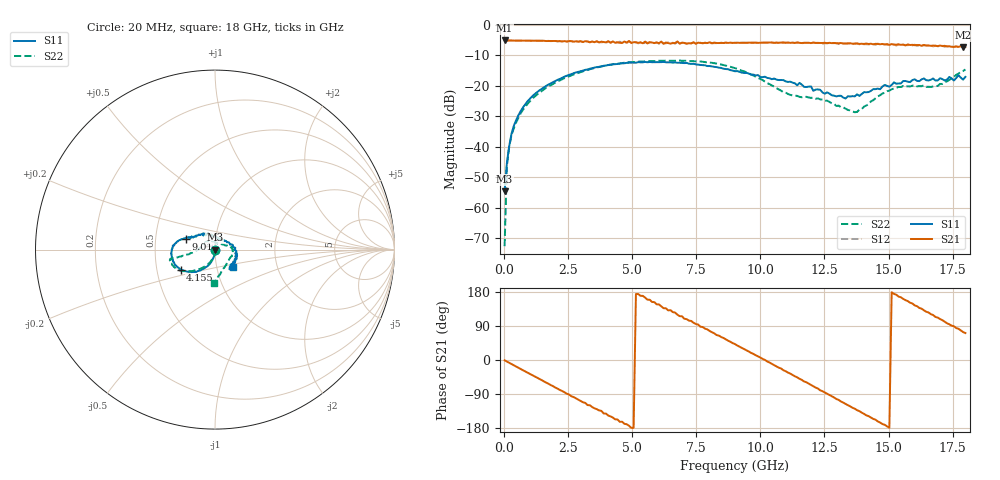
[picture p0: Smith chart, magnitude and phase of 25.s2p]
!Agilent Technologies,N5230A,US43500223,A.07.50.48
!Agilent N5230A: A.07.50.48
!Date: Wednesday, January 13, 2016 12:40:09
!Correction: S11(Full 2 Port(1,2))
!S21(Full 2 Port(1,2))
!S12(Full 2 Port(1,2))
!S22(Full 2 Port(1,2))
!S2P File: Measurements: S11, S21, S12, S22:
# Hz S  dB  R 50
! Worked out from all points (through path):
!   201 points, 20 MHz to 18 GHz, reference 50 ohm
!   highest |S21| = -5.16 dB at 20 MHz (marker M1); lowest = -7.4 dB at 17.91 GHz (marker M2)
!   group delay of S21, straight-line fit = 99.6 ps
!   lowest |S11| = -54.5 dB at 20 MHz (marker M3), VSWR 1.00, Z = 49.8 - j0.109 ohm
!   |S11| at or under -10 dB: start of sweep to end of sweep
!   |S22| runs from -72.5 to -11.7 dB; largest |S21 - S12| = 0.042
!   S11 on the Smith chart (normalised r, x): 20 MHz: 1.00, -0.00; 4.155 GHz: 0.66, -0.16; 9.01 GHz: 0.72, +0.09; 18 GHz: 1.20, -0.24
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2e7  -54.55 -144.2  -5.16 -0.8  -5.17 -0.9  -72.52 -110.8
1.099e8  -45.22 -107.3  -5.18 -4.1  -5.18 -4.1  -46.16 -82.0
2.897e8  -35.69 -91.2  -5.19 -10.8  -5.20 -10.8  -36.11 -87.4
4.695e8  -31.26 -95.9  -5.21 -17.2  -5.21 -17.4  -32.03 -93.7
9.19e8  -25.03 -103.3  -5.23 -33.6  -5.25 -33.8  -25.88 -103.0
1.3685e9  -21.57 -109.7  -5.29 -49.9  -5.29 -50.2  -22.32 -111.8
2.3574e9  -17.01 -124.9  -5.37 -85.2  -5.42 -85.5  -17.49 -127.2
3.0766e9  -15.04 -134.9  -5.69 -111.5  -5.61 -112.0  -15.25 -136.3
4.1554e9  -13.09 -149.8  -5.91 -148.9  -5.88 -150.2  -13.10 -147.9
4.8746e9  -12.43 -159.3  -5.33 -173.6  -5.57 -173.4  -12.29 -154.1
6.0433e9  -12.27 -173.6  -6.06 146.5  -6.28 143.8  -11.81 -162.9
7.3918e9  -12.82 172.7  -5.76 98.2  -5.83 97.9  -11.94 -168.2
9.01e9  -15.24 159.2  -5.92 42.0  -5.93 39.8  -14.24 -168.6
1.04484e10  -17.85 145.9  -5.81 -10.3  -5.90 -12.5  -19.90 -177.7
1.20666e10  -21.66 109.3  -5.83 -69.1  -5.97 -71.6  -23.90 136.2
1.36848e10  -23.47 52.9  -6.15 -128.6  -6.31 -130.5  -28.67 69.9
1.50333e10  -20.32 10.1  -6.62 -178.8  -6.62 177.6  -21.58 11.2
1.66515e10  -18.02 -24.8  -6.93 121.0  -6.74 117.7  -20.39 -35.1
1.75505e10  -18.28 -44.8  -7.26 89.2  -7.33 83.6  -17.07 -78.1
1.77303e10  -16.56 -46.1  -7.27 82.4  -7.26 77.1  -16.02 -85.2
1.79101e10  -17.98 -49.3  -7.44 73.7  -7.29 70.9  -15.16 -89.1
1.8e10  -17.08 -44.2  -7.28 71.1  -7.55 66.9  -14.67 -91.2
